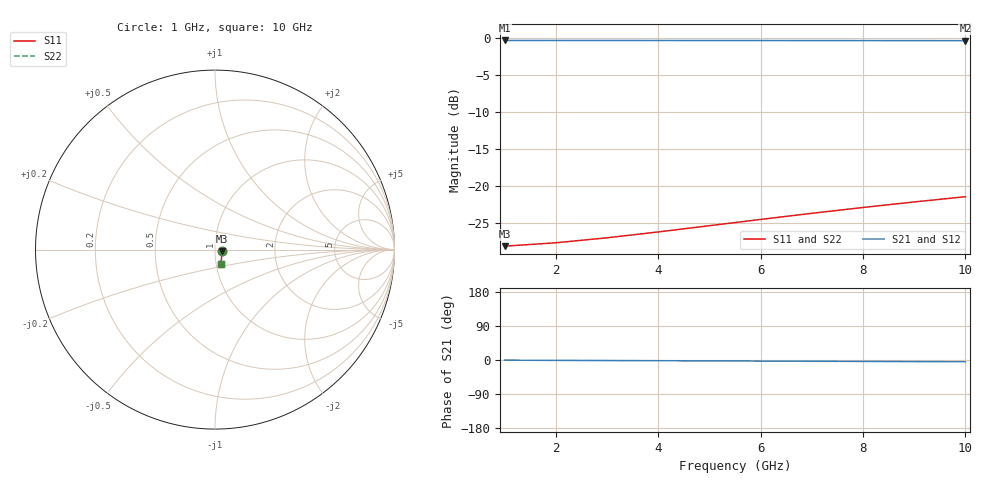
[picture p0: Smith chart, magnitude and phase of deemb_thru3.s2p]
! Created Tue Nov  2 11:41:51 2021
# hz S ma R 50
! 2 Port Network Data from SP1.SP block
! freq  magS11  angS11  magS21  angS21  magS12  angS12  magS22  angS22
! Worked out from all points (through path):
!   10 points, 1 GHz to 10 GHz, reference 50 ohm
!   highest |S21| = -0.34 dB at 1 GHz (marker M1); lowest = -0.4 dB at 10 GHz (marker M2)
!   lowest |S11| = -28.1 dB at 1 GHz (marker M3), VSWR 1.08, Z = 54 - j0.851 ohm
!   |S11| at or under -10 dB: start of sweep to end of sweep
!   |S22| runs from -28.1 to -21.5 dB; largest |S21 - S12| = 0
1e9  0.0392 -11.6  0.9615 -0.5  0.9615 -0.5  0.0392 -11.6
2e9  0.04132 -22.4  0.9614 -0.9  0.9614 -0.9  0.04132 -22.4
3e9  0.04464 -31.9  0.9613 -1.4  0.9613 -1.4  0.04464 -31.9
4e9  0.04891 -40.0  0.9611 -1.9  0.9611 -1.9  0.04891 -40.0
5e9  0.0539 -46.8  0.9608 -2.3  0.9608 -2.3  0.0539 -46.8
6e9  0.05942 -52.4  0.9605 -2.8  0.9605 -2.8  0.05942 -52.4
7e9  0.06534 -57.1  0.9601 -3.3  0.9601 -3.3  0.06534 -57.1
8e9  0.07156 -61.1  0.9596 -3.7  0.9596 -3.7  0.07156 -61.1
9e9  0.07799 -64.6  0.9591 -4.2  0.9591 -4.2  0.07799 -64.6
1e10  0.0846 -67.5  0.9586 -4.7  0.9586 -4.7  0.0846 -67.5
